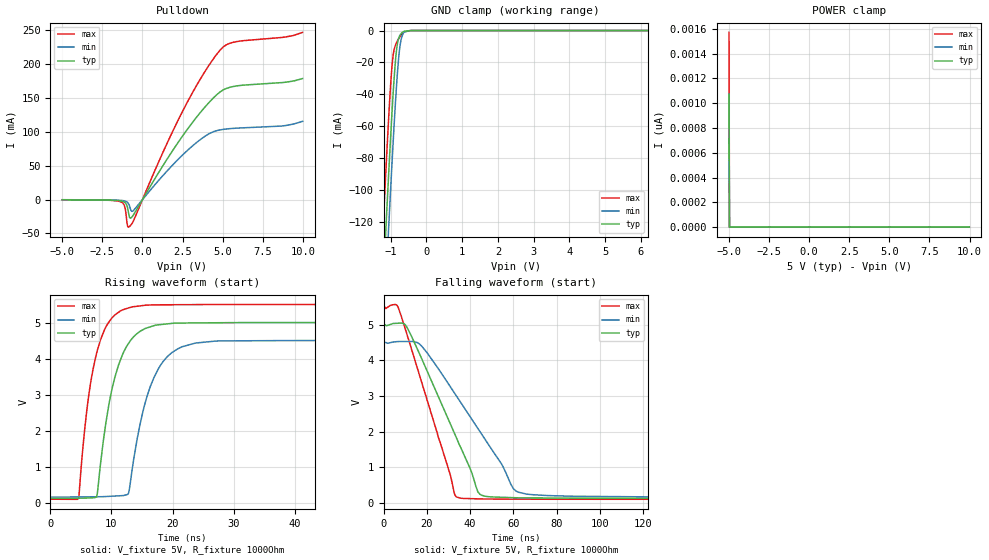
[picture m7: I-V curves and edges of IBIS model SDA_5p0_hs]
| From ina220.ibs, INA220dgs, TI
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|   Model
[Model]   SDA_5p0_hs
Model_type   I/O_open_drain
Polarity   Non-Inverting
Enable   Active-Low
Vinl = 1.5
Vinh = 3.5
Vmeas = 2.5
Vref = 5
Cref = 1pF
Rref = 1000
|   typ   min   max
C_comp   2.1193190E-12   1.8449300E-12 2.3639330E-12
[Voltage Range]   5   4.5   5.5
[Temperature Range]   27   85   -40
[Pullup Reference]   5   4.5   5.5
[Pulldown Reference]   -0   -0   -0
[Power Clamp Reference]   5   4.5   5.5
[GND Clamp Reference]   -0   -0   -0
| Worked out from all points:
|   slope of the pulldown table from 0 to 0.75 V, typ, clamps not added: 25.1 ohm
|   GND clamp passes 1 mA (typ) near -0.66 V on its own axis
|   falling waveform, V_fixture 5V, R_fixture 1000Ohm: 20-80 % time 21.2ns typ, 28.3ns min, 16.4ns max; typ from 5 V to 0.12 V
|   rising waveform, V_fixture 5V, R_fixture 1000Ohm: 20-80 % time 3.39ns typ, 3.95ns min, 2.89ns max; typ from 0.12 V to 5 V
[Pulldown]
|   Voltage   I(typ)   I(min)   I(max)
-5V       -196.2uA   -136.7uA   -251uA
-1.25V    -2.441mA   -1.382mA   -4.492mA
-1.085V   -4.401mA   -2.153mA   -12.11mA
-965mV    -9.014mA   -3.462mA   -34.28mA
-830mV    -24.29mA   -7.959mA   -40.07mA
-710mV    -26.92mA   -16.23mA   -37.21mA
-575mV    -23.01mA   -16.32mA   -31.97mA
2.53V     94.89mA    66.52mA    131.7mA
4V        139.4mA    95.09mA    193mA
4.84V     158.9mA    102.9mA    220.6mA
5.68V     167.1mA    105.2mA    232.4mA
9.985V    178.8mA    115.5mA    247mA
[GND Clamp]
|   Voltage   I(typ)   I(min)   I(max)
-5V       -2.019A    -2.05A     -1.986A
-1.25V    -176mA     -210.3mA   -138.9mA
-1.145V   -127.9mA   -162mA     -91.29mA
-1.1V     -107.8mA   -141.6mA   -71.72mA
-1.055V   -88.14mA   -121.6mA   -53.09mA
-965mV    -51.09mA   -82.87mA   -22.18mA
-920mV    -34.59mA   -64.52mA   -13.48mA
-860mV    -16.84mA   -41.85mA   -8.642mA
-800mV    -6.709mA   -22.67mA   -5.926mA
-740mV    -2.824mA   -9.434mA   -3.68mA
-620mV    -430.2uA   -885.3uA   -725.2uA
9.985V    0A         0A         0A
[POWER Clamp]
|   Voltage   I(typ)   I(min)   I(max)
-5V       1.074nA    713.1pA    1.571nA
-4.97V    0A         0A         0A
-4.955V   0A         0A         0A
9.985V    0A         0A         0A
[Ramp]
R_load = 1000
|   typ   min   max
dV/dt_r   2.92774/3.37279e-09   2.60948/3.92759e-09   3.24271/2.87134e-09
dV/dt_f   2.92774/2.12298e-08   2.60946/2.8327e-08   3.24271/1.64173e-08
[Falling Waveform]
V_fixture = 5V
V_fixture_min = 4.5V
V_fixture_max = 5.5V
R_fixture = 1000Ohm
C_fixture = 0F
|   Time   V(typ)   V(min)   V(max)
0s        5V         4.5V       5.5V
6.811ns   5.042V     4.527V     5.477V
10.7ns    4.936V     4.529V     4.744V
17.52ns   4.056V     4.404V     3.396V
32.93ns   1.924V     3.064V     220.1mV
35.24ns   1.598V     2.852V     131.2mV
44.47ns   238.7mV    2.003V     108mV
59.93ns   142.3mV    399.3mV    101.4mV
68.06ns   135.7mV    229.9mV    99.55mV
500ns     120.4mV    150.9mV    95.49mV
[Rising Waveform]
V_fixture = 5V
V_fixture_min = 4.5V
V_fixture_max = 5.5V
R_fixture = 1000Ohm
C_fixture = 0F
|   Time   V(typ)   V(min)   V(max)
0s        120.4mV    150.9mV    95.49mV
4.618ns   124mV      158.6mV    116.7mV
6.004ns   128.4mV    160.9mV    2.599V
7.584ns   166.2mV    163.5mV    4.152V
9.822ns   2.934V     176.7mV    5.067V
12.79ns   4.417V     261.2mV    5.403V
15.58ns   4.838V     2.808V     5.48V
19.9ns    4.976V     4.166V     5.493V
27.89ns   4.994V     4.49V      5.5V
500ns     5V         4.5V       5.5V
